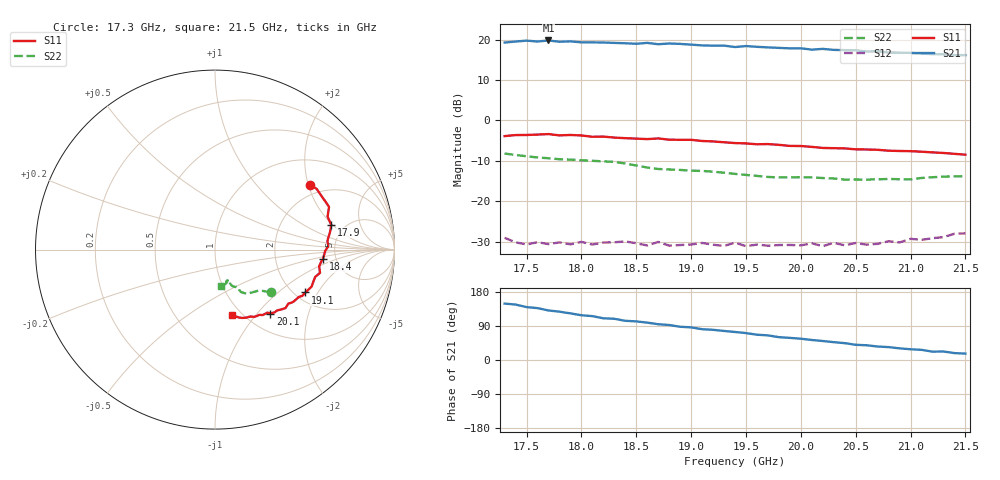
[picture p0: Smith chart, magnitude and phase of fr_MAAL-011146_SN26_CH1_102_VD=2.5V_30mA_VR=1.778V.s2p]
!Typical measured data - probed
!Date: Friday, August 19, 2022 11:59:35
!Correction: S11(Full 2 Port(1,2))
!S21(Full 2 Port(1,2))
!S12(Full 2 Port(1,2))
!S22(Full 2 Port(1,2))
!S2P File: Measurements: S11, S21, S12, S22:
# Hz S  dB  R 50
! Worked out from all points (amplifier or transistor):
!   43 points, 17.3 GHz to 21.5 GHz, reference 50 ohm
!   highest |S21| = 19.8 dB at 17.7 GHz (marker M1)
!   |S21| within 3 dB of that: start of sweep to 20.8 GHz
!   unconditionally stable (mu >= 1): start of sweep to end of sweep
!   at 18 GHz: K = 1.11, MAG = 22.7 dB, |S12| = -30.1 dB
!   at 19.4 GHz: K = 1.57, MAG = 19.8 dB, |S12| = -30.2 dB
!   at 21.5 GHz: K = 1.76, MAG = 17.0 dB, |S12| = -27.9 dB
!   S11 on the Smith chart (normalised r, x): 17.3 GHz: 1.68, +2.05; 17.9 GHz: 3.90, +1.93; 18.4 GHz: 3.93, -0.66; 19.1 GHz: 2.27, -1.57; 20.1 GHz: 1.28, -1.18; 21.5 GHz: 0.90, -0.77
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1.73e10  -3.87 34.3  19.28 148.9  -29.05 -46.2  -8.19 -37.4
1.74e10  -3.61 30.9  19.54 146.3  -30.17 -49.4  -8.54 -38.9
1.75e10  -3.59 28.9  19.76 139.6  -30.70 -43.6  -8.86 -40.0
1.76e10  -3.49 24.3  19.54 136.9  -30.13 -48.3  -9.16 -41.2
1.77e10  -3.37 20.5  19.81 130.7  -30.61 -43.3  -9.36 -42.4
1.79e10  -3.59 12.2  19.57 123.0  -30.66 -46.0  -9.69 -45.1
1.8e10  -3.72 9.4  19.35 118.1  -30.06 -44.4  -9.85 -46.8
1.83e10  -4.24 -0.8  19.20 108.8  -30.15 -48.2  -10.26 -53.3
1.84e10  -4.38 -5.1  19.11 103.4  -29.95 -44.1  -10.66 -55.9
1.86e10  -4.61 -9.1  19.20 98.6  -30.95 -49.0  -11.65 -59.0
1.87e10  -4.44 -12.5  18.88 94.4  -30.07 -47.2  -12.01 -58.6
1.88e10  -4.76 -15.3  19.05 92.3  -30.98 -48.2  -12.13 -58.8
1.91e10  -5.08 -25.4  18.57 81.3  -30.32 -48.0  -12.49 -61.4
1.94e10  -5.60 -33.5  18.17 73.9  -30.25 -53.0  -13.22 -65.4
1.95e10  -5.68 -34.6  18.42 71.1  -31.12 -51.0  -13.48 -65.6
1.98e10  -6.04 -41.8  17.97 60.3  -30.84 -48.5  -14.11 -65.7
2.01e10  -6.54 -49.2  17.53 52.8  -30.41 -51.2  -14.11 -66.6
2.05e10  -7.15 -55.9  17.37 40.1  -30.33 -53.0  -14.61 -67.9
2.08e10  -7.49 -61.9  16.80 34.0  -29.89 -51.5  -14.48 -69.9
2.12e10  -7.90 -70.3  16.42 22.0  -29.15 -51.7  -14.06 -71.3
2.13e10  -8.04 -71.5  16.39 22.5  -28.87 -53.5  -13.89 -74.7
2.15e10  -8.47 -75.1  16.17 16.9  -27.95 -55.7  -13.79 -81.2
